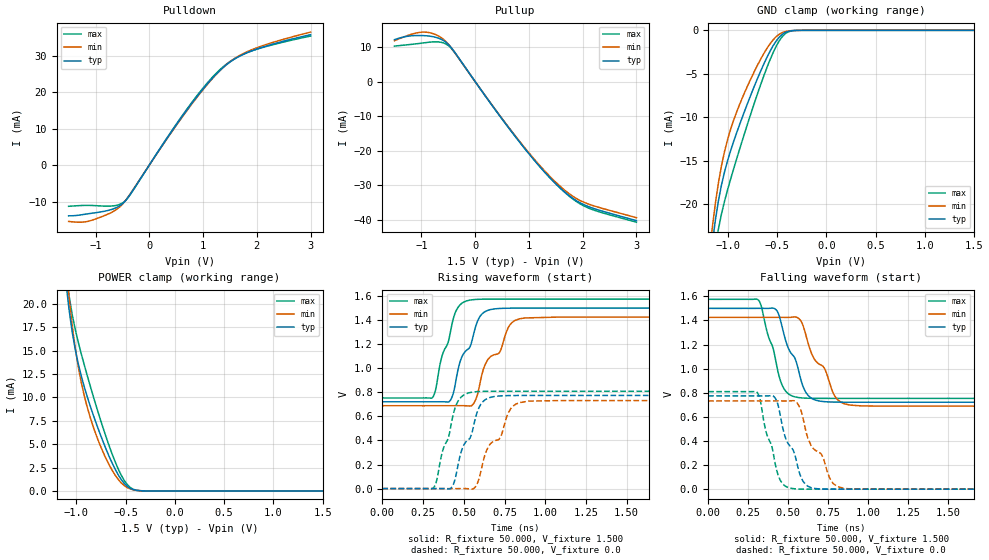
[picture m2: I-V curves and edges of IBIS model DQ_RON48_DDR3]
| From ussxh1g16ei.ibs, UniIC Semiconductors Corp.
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|   Model DQ_RON48_DDR3
[Model] DQ_RON48_DDR3
Model_type I/O
Vinl =  0.615V
Vinh =  0.885V
Vmeas =  0.750V
Rref =  50.000
Vref =  0.750V
C_comp   1.232pF   1.219pF   1.235pF
[Model Spec]
Vinh   0.885V   0.847V   0.922V
Vinl   0.615V   0.577V   0.652V
Vmeas   0.750V   0.712V   0.787V
Vref   0.750V   0.712V   0.787V
Rref   50.000   NA   NA
[Temperature Range]   25.000   95.000   -40.000
[Voltage Range]   1.500V   1.425V   1.575V
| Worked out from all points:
|   slope of the pulldown table from 0 to 0.225 V, typ, clamps not added: 44.5 ohm
|   slope of the pullup table from 0 to 0.225 V, typ, clamps not added: 45.5 ohm
|   GND clamp passes 1 mA (typ) near -0.49 V on its own axis
|   POWER clamp passes 1 mA (typ) near -0.53 V on its own axis
|   rising waveform, R_fixture 50.000, V_fixture 1.500: 20-80 % time 123ps typ, 162ps min, 95.8ps max; typ from 0.721 V to 1.5 V
|   rising waveform, R_fixture 50.000, V_fixture 0.0: 20-80 % time 120ps typ, 155ps min, 94.4ps max; typ from 0 V to 0.774 V
|   falling waveform, R_fixture 50.000, V_fixture 1.500: 20-80 % time 124ps typ, 159ps min, 97.7ps max; typ from 1.5 V to 0.721 V
|   falling waveform, R_fixture 50.000, V_fixture 0.0: 20-80 % time 117ps typ, 151ps min, 90ps max; typ from 0.774 V to 0 V
[Pulldown]
|Voltage   I(typ)   I(min)   I(max)
-1.5V     -13.93mA   -15.46mA   -11.31mA
-1.086V   -13.25mA   -15.22mA   -11.07mA
-718mV    -12.25mA   -13.11mA   -11.25mA
-488mV    -10.47mA   -10.56mA   -10.3mA
-350mV    -7.917mA   -7.8mA     -8.022mA
294mV     6.573mA    6.465mA    6.684mA
754mV     16.22mA    16.03mA    16.46mA
1.076V    22.24mA    22.08mA    22.49mA
1.352V    26.51mA    26.48mA    26.71mA
1.582V    29.08mA    29.2mA     29.19mA
1.904V    31.36mA    31.66mA    31.33mA
3V        35.8mA     36.51mA    35.43mA
[Pullup]
|Voltage   I(typ)   I(min)   I(max)
-1.5V     12.11mA    11.8mA     10.24mA
-1.14V    13.26mA    13.86mA    10.82mA
-910mV    13.22mA    14.27mA    11.26mA
-680mV    12.53mA    13.15mA    11.45mA
-496mV    10.71mA    10.78mA    10.38mA
-358mV    7.998mA    7.944mA    7.888mA
746mV     -15.88mA   -15.69mA   -15.78mA
1.16V     -23.82mA   -23.51mA   -23.76mA
1.528V    -29.95mA   -29.51mA   -29.99mA
1.804V    -33.59mA   -33.02mA   -33.79mA
2.034V    -35.66mA   -34.95mA   -36.03mA
3V        -40.2mA    -39.34mA   -40.64mA
[GND_clamp]
|Voltage   I(typ)   I(min)   I(max)
-1.5V     -77.15mA   -73.99mA   -84.26mA
-1.159V   -24.58mA   -22.75mA   -27.74mA
-1.128V   -21.88mA   -19.96mA   -25.03mA
-1.097V   -19.64mA   -17.59mA   -22.88mA
-1.066V   -17.82mA   -15.61mA   -21.14mA
-1.004V   -15mA      -12.58mA   -18.36mA
-880mV    -10.79mA   -8.48mA    -13.61mA
-632mV    -3.776mA   -2.594mA   -5.119mA
-477mV    -756.2uA   -431.9uA   -1.164mA
-415mV    -225.6uA   -131.2uA   -354.1uA
-322mV    -19.15uA   -14.82uA   -24.1uA
1.5V      0A         0A         0A
[POWER_clamp]
|Voltage   I(typ)   I(min)   I(max)
-1.5V     91.1mA     92.64mA    94.46mA
-1.104V   22.28mA    23.97mA    23.43mA
-1.073V   19.41mA    20.63mA    20.89mA
-1.042V   17.07mA    17.76mA    18.91mA
-980mV    13.62mA    13.3mA     15.93mA
-918mV    11.11mA    10.16mA    13.45mA
-856mV    9.013mA    7.787mA    11.15mA
-670mV    3.78mA     2.864mA    4.931mA
-577mV    1.775mA    1.269mA    2.414mA
-484mV    502.3uA    362.1uA    693.5uA
-329mV    12.96uA    15.92uA    9.805uA
1.5V      0A         0A         0A
[Ramp]
| variable   typ   min   max
dV/dt_r   0.464/0.120n   0.439/0.155n   0.485/94.236p
dV/dt_f   0.467/0.124n   0.442/0.159n   0.493/97.663p
R_load = 50.000
[Rising Waveform]
R_fixture= 50.000
V_fixture= 1.500
V_fixture_min= 1.425
V_fixture_max= 1.575
|time   V(typ)   V(min)   V(max)
0s        721.4mV    688.7mV    753.1mV
312ps     721.4mV    688.7mV    764.1mV
410ps     722.5mV    688.7mV    1.249V
444ps     841.2mV    688.7mV    1.449V
480ps     1.066V     688.9mV    1.531V
537ps     1.175V     686.4mV    1.566V
581ps     1.38V      768.8mV    1.572V
621ps     1.462V     996mV      1.574V
843ps     1.5V       1.411V     1.575V
3ns       1.5V       1.425V     1.575V
[Rising Waveform]
R_fixture= 50.000
V_fixture= 0.0
V_fixture_min= 0.0
V_fixture_max= 0.0
|time   V(typ)   V(min)   V(max)
0s        156.4nV    636.5nV    65.49nV
314ps     -4.582uV   9.103uV    5.664mV
415ps     -1.551mV   7.136uV    479.9mV
451ps     104.5mV    -25.85uV   687.6mV
491ps     334.9mV    455.4uV    769.1mV
539ps     422.2mV    -3.629mV   798.3mV
585ps     646.3mV    49.33mV    806mV
628ps     735.1mV    272.6mV    808.2mV
840ps     773.7mV    713.8mV    809.1mV
3ns       774mV      731.8mV    809.2mV
[Falling Waveform]
R_fixture= 50.000
V_fixture= 1.500
V_fixture_min= 1.425
V_fixture_max= 1.575
|time   V(typ)   V(min)   V(max)
0s        1.5V       1.425V     1.575V
315ps     1.5V       1.425V     1.568V
417ps     1.497V     1.425V     1.106V
459ps     1.367V     1.425V     874.9mV
551ps     1.058V     1.428V     763.4mV
635ps     765.6mV    1.169V     754.2mV
730ps     725.8mV    997.8mV    753.2mV
795ps     722.3mV    767mV      753.1mV
854ps     721.6mV    707.5mV    753.1mV
3ns       721.4mV    688.7mV    753.1mV
[Falling Waveform]
R_fixture= 50.000
V_fixture= 0.0
V_fixture_min= 0.0
V_fixture_max= 0.0
|time   V(typ)   V(min)   V(max)
0s        774mV      731.8mV    809.2mV
308ps     773.9mV    731.8mV    800.5mV
422ps     749.9mV    731.8mV    193.8mV
515ps     352.7mV    732.6mV    8.24mV
571ps     135.4mV    683mV      1.186mV
616ps     32.03mV    457.1mV    244uV
711ps     1.384mV    284.7mV    8.772uV
771ps     187.2uV    66.57mV    1.231uV
859ps     10.1uV     4.525mV    236.7nV
3ns       261.9nV    757.2nV    149.9nV
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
